(* Logix 5000 DataType export; software revision 16.04 *)

TYPE AKD_Control :   // Send Explicit Message
STRUCT
   Load_Data_Start_Profile : BOOL;   // Load Command Data / Start Profile Move
   Start_Block : BOOL;   // Execute Command block or block chain
   Incremental : BOOL;   // Incremental Position (0=Absolute, 1=Incremental)
   Direction : BOOL;   // Direction in Velocity Mode (0=Reverse, 1=Forward)
   Smooth_Stop : BOOL;   // Smooth / Controlled Stop w/ Deceleration
   Hard_Stop : BOOL;   // Hard / Immediate Stop
   Reg_Arm : BOOL;   // Arm the Registration Input
   Enable : BOOL;   // Enable Output
END_STRUCT
END_TYPE
